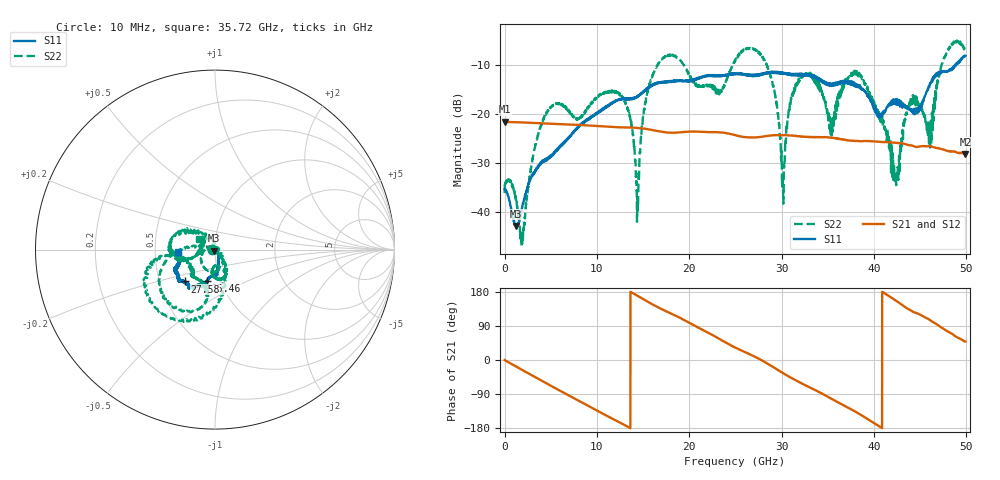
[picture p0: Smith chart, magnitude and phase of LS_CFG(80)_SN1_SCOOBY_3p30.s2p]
!Keysight Technologies,N5245B,MY58422026,A.13.80.08
!Date: Thursday, March 19, 2020 23:52:07
!Correction: S11(Full 2 Port(1,2))
!S21(Full 2 Port(1,2))
!S12(Full 2 Port(1,2))
!S22(Full 2 Port(1,2))
!S2P File: Measurements: S11, S21, S12, S22:
# Hz S DB R 50.0
!freq dBS11 angS11 dBS21 angS21 dBS12 angS12 dBS22 angS22
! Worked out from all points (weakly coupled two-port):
!   4991 points, 10 MHz to 49.91 GHz, reference 50 ohm
!   highest |S21| = -21.66 dB at 10 MHz (marker M1); lowest = -28.2 dB at 49.91 GHz (marker M2)
!   lowest |S11| = -42.9 dB at 1.23 GHz (marker M3), VSWR 1.01, Z = 49.5 - j0.533 ohm
!   |S11| at or under -10 dB: start of sweep to 48.88 GHz; 48.94794 GHz to 48.98193 GHz (33.98 MHz wide, 0.0694 % of centre)
!   |S22| runs from -47.0 to -5.1 dB; largest |S21 - S12| = 0.00081
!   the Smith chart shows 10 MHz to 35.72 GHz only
!   S11 on the Smith chart (normalised r, x): 10 MHz: 0.97, -0.01; 15.46 GHz: 0.86, -0.31; 27.58 GHz: 0.67, -0.25; 35.72 GHz: 0.66, -0.02
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1e7  -35.35 -170.5  -21.66 -0.2  -21.65 -0.3  -36.18 176.6
1.23e9  -42.90 -131.2  -21.75 -16.9  -21.75 -16.9  -37.47 -99.3
1.94e9  -38.81 -67.5  -21.80 -26.6  -21.79 -26.5  -45.60 17.9
4.78e9  -28.84 -56.0  -22.05 -64.8  -22.04 -64.8  -19.23 -130.7
8.33e9  -22.26 -75.9  -22.34 -111.8  -22.33 -111.8  -20.59 -92.1
1.261e10  -16.97 -85.7  -22.80 -166.5  -22.80 -166.4  -16.32 -66.2
1.438e10  -16.48 -98.5  -22.91 169.7  -22.90 169.8  -38.07 -120.0
1.546e10  -14.89 -104.9  -23.17 154.5  -23.16 154.5  -15.45 175.8
1.665e10  -13.77 -103.9  -23.58 138.8  -23.57 138.8  -9.84 -158.4
2.496e10  -11.92 -124.8  -24.36 33.0  -24.35 33.3  -9.29 -168.1
2.758e10  -12.24 -133.5  -24.78 2.9  -24.78 3.1  -7.71 -109.0
3.015e10  -11.75 -143.1  -24.41 -34.3  -24.42 -34.0  -34.21 37.7
3.125e10  -11.91 -147.9  -24.51 -49.9  -24.51 -49.5  -15.38 138.3
3.328e10  -12.25 -156.1  -24.77 -75.2  -24.77 -74.8  -12.19 -173.8
3.572e10  -13.80 -175.4  -25.01 -106.5  -24.94 -106.0  -19.99 150.0
3.816e10  -14.56 173.7  -25.59 -138.5  -25.54 -138.6  -11.37 -174.9
4.16e10  -18.11 105.4  -25.83 169.2  -25.85 169.2  -25.22 71.8
4.245e10  -17.27 103.1  -25.96 155.6  -25.98 155.5  -34.14 -176.0
4.39e10  -19.13 75.5  -26.43 132.2  -26.45 132.3  -17.58 -32.2
4.601e10  -14.52 9.0  -26.59 106.4  -26.61 106.5  -23.11 114.6
4.771e10  -11.37 6.3  -27.44 79.2  -27.45 79.4  -8.18 -79.6
4.991e10  -8.21 -14.5  -28.23 48.6  -28.26 48.7  -7.32 -14.9
